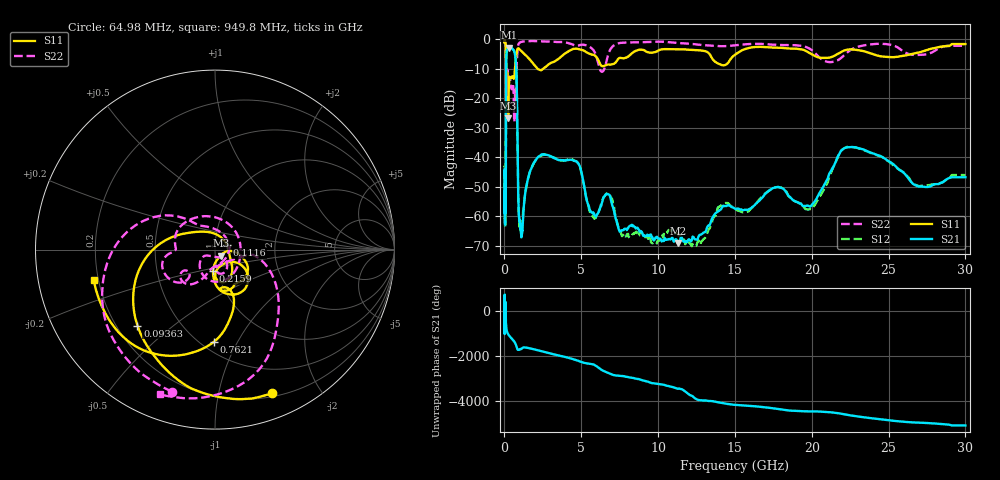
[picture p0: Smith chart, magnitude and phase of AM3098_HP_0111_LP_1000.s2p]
! Date/Time: Thu, Feb 28, 2019 8:38 AM
! Network Analyzer: Agilent Technologies E8364B Rev: A.07.50.67
! Sweep from 0.010 to 30.000 GHz, 1601 Points, Sweep Type: LOG
! Power Supply: 5.023 V, 0.002 A
# Hz S DB R 50
!freq MagS11 AngS11 MagS21 AngS21 MagS12 AngS12 MagS22 AngS22
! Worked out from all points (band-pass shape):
!   1601 points, 10 MHz to 30 GHz, reference 50 ohm
!   highest |S21| = -2.78 dB at 297.5 MHz (marker M1); lowest = -69.1 dB at 11.31 GHz (marker M2)
!   |S21| within 3 dB of the highest: 121.7 MHz to 707.1 MHz (585.3 MHz wide, 141 % of centre)
!   lowest |S11| = -26.8 dB at 239.9 MHz (marker M3), VSWR 1.10, Z = 53.1 - j3.53 ohm
!   |S11| at or under -10 dB: 102.2 MHz to 682.9 MHz (580.7 MHz wide, 148 % of centre); 2.164 GHz to 2.518 GHz (353.8 MHz wide, 15.1 % of centre)
!   |S22| runs from -28.0 to -0.5 dB; largest |S21 - S12| = 0.013
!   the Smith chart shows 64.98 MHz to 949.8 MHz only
!   S11 on the Smith chart (normalised r, x): 64.98 MHz: 0.23, -1.45; 93.63 MHz: 0.28, -0.38; 111.6 MHz: 1.14, +0.06; 215.9 MHz: 0.95, -0.23; 762.1 MHz: 0.58, -0.81; 949.8 MHz: 0.18, -0.12
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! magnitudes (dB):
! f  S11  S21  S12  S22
! 10 MHz  -0.3  -46.0  -44.2  -0.7
! 38.04 MHz  -0.5  -60.4  -61.3  -0.9
! 64.98 MHz  -1.3  -50.8  -52.4  -1.7
! 77.81 MHz  -1.8  -56.5  -54.6  -2.3
! 93.63 MHz  -4.4  -38.1  -38.3  -4.8
! 111.6 MHz  -23.0  -8.6  -8.6  -20.0
! 144.7 MHz  -20.0  -3.9  -3.9  -14.3
! 215.9 MHz  -18.3  -3.1  -3.0  -11.7
! 239.9 MHz  -26.8  -2.9  -2.8  -12.7
! 297.5 MHz  -14.8  -2.8  -2.7  -12.8
! 550.5 MHz  -12.7  -3.4  -3.4  -15.0
! 639.6 MHz  -12.7  -4.1  -4.0  -28.0
! 762.1 MHz  -5.8  -9.5  -9.4  -18.1
! 949.8 MHz  -3.1  -60.6  -60.6  -1.3
! 1.126 GHz  -4.0  -66.0  -65.1  -0.8
! 2.084 GHz  -9.6  -40.6  -40.5  -0.6
! 4.663 GHz  -3.1  -41.3  -41.3  -2.1
! 7.926 GHz  -6.1  -64.3  -66.7  -1.0
! 11.31 GHz  -3.3  -69.1  -66.5  -1.2
! 19.9 GHz  -4.7  -56.7  -57.6  -3.3
! 22.67 GHz  -3.4  -36.5  -36.6  -3.2
! 30 GHz  -1.6  -46.8  -46.0  -2.1
